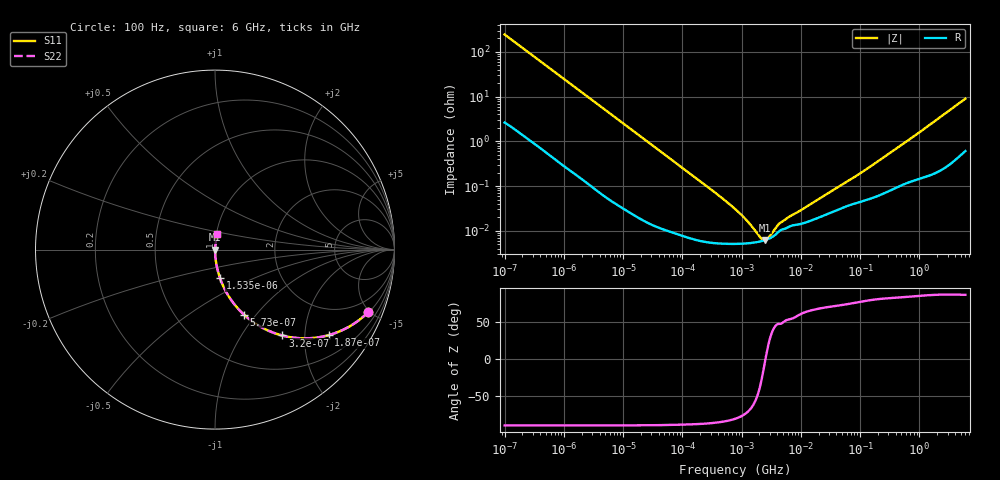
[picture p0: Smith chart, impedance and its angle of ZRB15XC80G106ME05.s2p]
!Murata Part Number: ZRB15XC80G106ME05
!These Parameters are Measured in Series Mode Connection
!Data Generated on Jun 10, 2025
!  o--ll--o
!Port1  Port2
!  o------o
!Operation Temp=25[degC], DC Bias Voltage=0[V]
!Freq. Start=100[Hz] Stop=6[GHz] 401[Steps]
# Hz S RI R 50
!Freq.(Hz) S11(Real) S11(Imag) S21(Real) S21(Imag) S12(Real) S12(Imag) S22(Real) S22(Imag)
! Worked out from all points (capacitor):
!   401 points, 100 Hz to 6 GHz, reference 50 ohm
!   read as one part in series: C = 6.47 uF near 109 Hz
!   lowest |Z| = 6.18 mohm at 2.481 MHz (marker M1)
!   series resonance near 2.534 MHz, so ESL is about 610 pH
!   S11 on the Smith chart (normalised r, x): 100 Hz: 1.05, -4.90; 187 Hz: 1.03, -2.63; 320 Hz: 1.02, -1.55; 573 Hz: 1.01, -0.87; 1.535 kHz: 1.00, -0.33; 6 GHz: 1.01, +0.18
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100  0.8548 -0.347  0.1452 0.347  0.1452 0.347  0.8548 -0.347
187  0.6329 -0.4765  0.3671 0.4765  0.3671 0.4765  0.6329 -0.4765
320  0.3752 -0.4785  0.6248 0.4785  0.6248 0.4785  0.3752 -0.4785
573  0.1611 -0.362  0.8389 0.362  0.8389 0.362  0.1611 -0.362
897  0.0742 -0.2566  0.9258 0.2566  0.9258 0.2566  0.0742 -0.2566
1535  0.0276 -0.1582  0.9724 0.1582  0.9724 0.1582  0.0276 -0.1582
2008  0.0167 -0.1226  0.9833 0.1226  0.9833 0.1226  0.0167 -0.1226
6433  0.00199 -0.0392  0.998 0.0392  0.998 0.0392  0.00199 -0.0392
40335  0.000156 -0.00634  0.9998 0.00634  0.9998 0.00634  0.000156 -0.00634
302498  5.47e-05 -0.000846  0.9999 0.000846  0.9999 0.000846  5.47e-05 -0.000846
774597  5.09e-05 -0.000304  0.9999 0.000304  0.9999 0.000304  5.09e-05 -0.000304
1658239  5.46e-05 -8.92e-05  0.9999 8.92e-05  0.9999 8.92e-05  5.46e-05 -8.92e-05
1896632  5.63e-05 -5.99e-05  0.9999 5.99e-05  0.9999 5.99e-05  5.63e-05 -5.99e-05
2481164  6.17e-05 -4.2e-06  0.9999 4.2e-06  0.9999 4.2e-06  6.17e-05 -4.2e-06
3394479  7.43e-05 6.01e-05  0.9999 -6.01e-05  0.9999 -6.01e-05  7.43e-05 6.01e-05
4440638  0.000101 0.000109  0.9999 -0.000109  0.9999 -0.000109  0.000101 0.000109
6075234  0.00012 0.000158  0.9999 -0.000158  0.9999 -0.000158  0.00012 0.000158
1.555665e7  0.000173 0.00038  0.9998 -0.00038  0.9998 -0.00038  0.000173 0.00038
8.918374e7  0.000424 0.00168  0.9996 -0.00168  0.9996 -0.00168  0.000424 0.00168
3.124326e8  0.000808 0.00532  0.9992 -0.00532  0.9992 -0.00532  0.000808 0.00532
1.791126e9  0.00266 0.0276  0.9973 -0.0276  0.9973 -0.0276  0.00266 0.0276
6e9  0.0138 0.0878  0.9862 -0.0878  0.9862 -0.0878  0.0138 0.0878
